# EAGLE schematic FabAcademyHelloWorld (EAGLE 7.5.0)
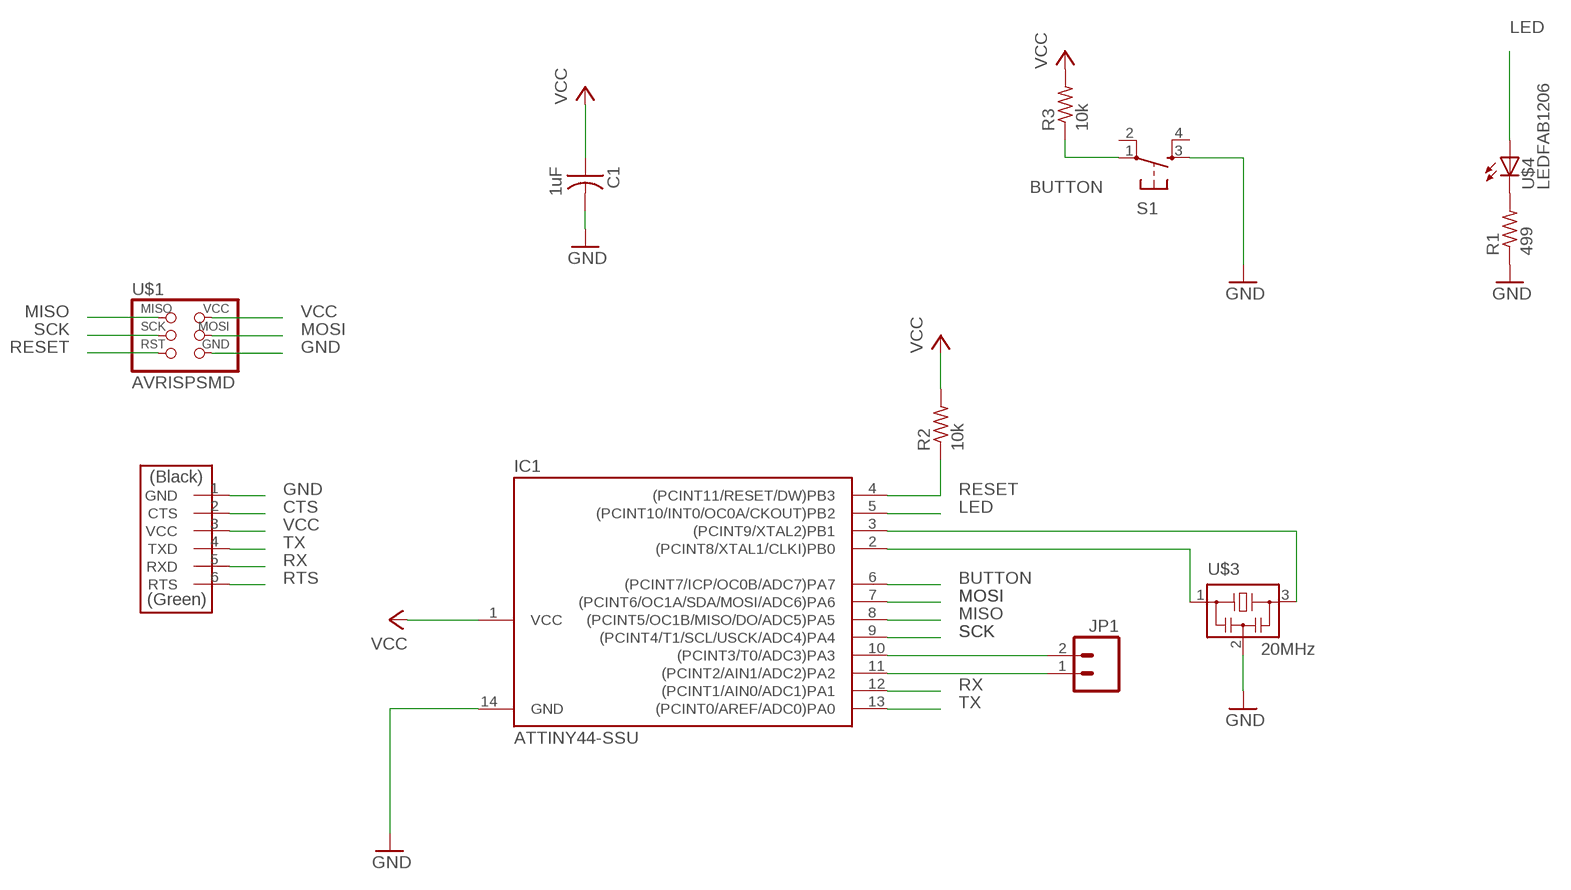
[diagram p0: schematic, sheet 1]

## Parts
C1  1uF  CAP-US1206FAB  [C1206FAB]
IC1  ATTINY44-SSU  [SOIC14]
JP1  M02PTH  [1X02]
R1  499  RES-US1206FAB  [R1206FAB]
R2  10k  RES-US1206FAB  [R1206FAB]
R3  10k  RES-US1206FAB  [R1206FAB]
S1  6MM_SWITCH6MM_SWITCH  [6MM_SWITCH]
U$1  AVRISPSMD  [2X03SMD]
U$2  FTDI-SMD-HEADER  [1X06SMD]
U$3  20MHz  RESONATOR  [EFOBM]
U$4  LEDFAB1206  [LED1206FAB]

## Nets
BUTTON: IC1.6((PCINT7/ICP/OC0B/ADC7)PA7) R3.1 S1.1(P)
CTS: U$2.2(CTS)
GND: C1.2 IC1.14(GND) R1.1 S1.3(S) U$1.6(GND) U$2.1(GND) U$3.2
LED: IC1.5((PCINT10/INT0/OC0A/CKOUT)PB2) U$4.1(A)
MISO: IC1.8((PCINT5/OC1B/MISO/DO/ADC5)PA5) U$1.1(MISO)
MOSI: IC1.7((PCINT6/OC1A/SDA/MOSI/ADC6)PA6) U$1.4(MOSI)
N$1: R1.2 U$4.2(C)
N$2: IC1.2((PCINT8/XTAL1/CLKI)PB0) U$3.1
N$3: IC1.11((PCINT2/AIN1/ADC2)PA2) JP1.1
N$4: IC1.10((PCINT3/T0/ADC3)PA3) JP1.2
N$9: IC1.3((PCINT9/XTAL2)PB1) U$3.3
RESET: IC1.4((PCINT11/RESET/DW)PB3) R2.1 U$1.5(RST)
RTS: U$2.6(RTS)
RX: IC1.12((PCINT1/AIN0/ADC1)PA1) U$2.5(RXD)
SCK: IC1.9((PCINT4/T1/SCL/USCK/ADC4)PA4) U$1.3(SCK)
TX: IC1.13((PCINT0/AREF/ADC0)PA0) U$2.4(TXD)
VCC: C1.1 IC1.1(VCC) R2.2 R3.2 U$1.2(VCC) U$2.3(VCC)
Unconnected: S1.2(P1) S1.4(S1)

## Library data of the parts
C1 = fablab:CAP-US
IC1 = fablab:ATTINY44
JP1 = SparkFun-Connectors:M02: Standard 2-pin 0.1" header. Use with
R1-R3 = fablab:RES-US: Resistor (US Symbol)
S1 = fablab:6MM_SWITCH: OMRON SWITCH
U$1 = fablab:AVRISP
U$2 = fablab:FTDI-SMD-HEADER
U$3 = fablab:RESONATOR
U$4 = fablab:LED: LED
